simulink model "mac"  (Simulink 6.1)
settings: Solver=ode45  StartTime=0.0  StopTime=10  RelTol=1e-3
undefined symbols (not defined in the file or in its folder): coef, Ft, juan2, mac_clk_wrapper, netlist, XFix
libraries: xbsIndex_r3 x9

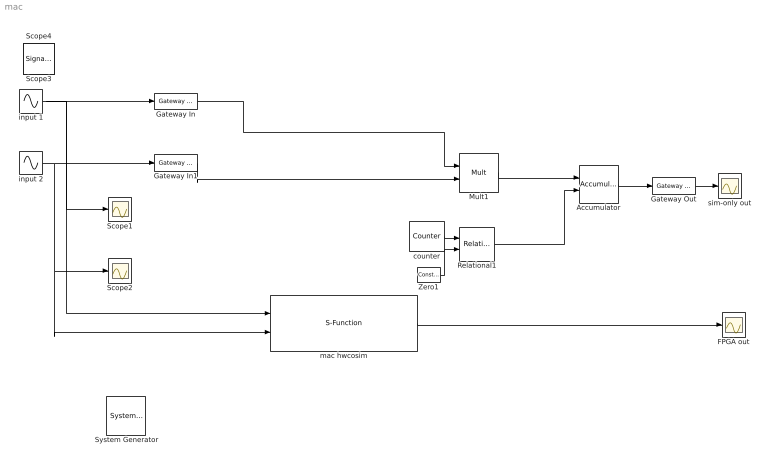
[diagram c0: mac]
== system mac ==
  " System Generator" : xbsIndex_r3/ System Generator  Tag=genX  xilinxfamily=Virtex2  part=xc2v1000  speed=-4  package=fg456  synthesis_tool=XST  directory=./netlist  testbench=off  simulink_period=1/2  sysclk_period=10  incr_netlist=off  trim_vbits=Everywhere in SubSystem  dbl_ovrd=According to Block Masks  core_generation=According to Block Masks  run_coregen=off  deprecated_control=off  eval_field=0
  Accumulator : xbsIndex_r3/Accumulator  n_bits=16  overflow=Wrap  operation=Add  scale=1  explicit_period=off  period=1  rst=on  hasbypass=off  en=off  dbl_ovrd=off  show_param=on  gen_core=off  use_rpm=on
  FPGA out : Scope
  Gateway In : xbsIndex_r3/Gateway In  arith_type="Signed  (2's comp)"  n_bits=8  bin_pt=6  quantization=Truncate  overflow=Wrap  period=1  timing_constraint=None  locs_specified=off  LOCs={}  needs_fixed_name=off  dbl_ovrd=off  show_param=off
  Gateway In1 : xbsIndex_r3/Gateway In  arith_type="Signed  (2's comp)"  n_bits=8  bin_pt=6  quantization=Truncate  overflow=Wrap  period=1  timing_constraint=None  locs_specified=off  LOCs={}  needs_fixed_name=off  dbl_ovrd=off  show_param=off
  Gateway Out : xbsIndex_r3/Gateway Out  output_type=Double  nbits=8  bin_pt=6  arith_type=Boolean  quantization=Truncate  overflow=Wrap  hdl_port=on  timing_constraint=None  locs_specified=off  LOCs={}  needs_fixed_name=off  show_param=off
  Mult1 : xbsIndex_r3/Mult  precision=Full  arith_type="Signed  (2's comp)"  n_bits=8  bin_pt=2  quantization=Truncate  overflow=Wrap  latency=2  explicit_period=on  period=1  en=off  dbl_ovrd=off  show_param=off  mult_type=Parallel  oversample=2  use_embedded=off  pipeline=on  use_rpm=on  placement_style=Rectangular Shape  gen_core=off
  Relational1 : xbsIndex_r3/Relational  mode=a=b  latency=0  explicit_period=on  period=-1  en=off  dbl_ovrd=off  show_param=off
  Scope1 : Scope
  Scope2 : Scope
  Zero1 : xbsIndex_r3/Constant  Priority=5  const=32  equ=P=C  arith_type=Unsigned  n_bits=5  bin_pt=0  opselect=C  inp2=PCIN>>17  opr=+  inp1=P  carry=CIN  iostate=0  explicit_period=off  period=Ft/length(coef)  dbl_ovrd=off
  counter : xbsIndex_r3/Counter  Priority=5  cnt_type=Count Limited  n_bits=5  bin_pt=0  arith_type=Unsigned  start_count=0  cnt_to=31  cnt_by_val=1  operation=Up  explicit_period=off  period=1  load_pin=off  rst=off  en=off  dbl_ovrd=off  show_param=off  use_rpm=on  gen_core=on
  input 1 : Sin  Amplitude=.5  Frequency=2*pi/23  Phase=pi/6  SampleTime=1
  input 2 : Sin  Amplitude=.5  Frequency=2*pi/23  Phase=pi/6  SampleTime=1
  mac hwcosim : S-Function  FunctionName=xlcosim  Parameters=sfcn_mwsv__  mask(Xilinx JTAG Hardware Co-Simulation){bitfileName=t:\juan2\netlist\mac_clk_wrapper.bit, clkSrc=Single Stepped, hasBufgmux=on, blkPeriod=0.5, IRLengths=[8,6], bscanPos=2, prtSignalType=XFix, prtNames={'gateway_in','gateway_in1','gateway_out'}, prtTypes={'Fix_8_6','Fix_8_6','Fix_16_12'}, prtDirs=[0,0,1], prtDataRates=[2,2,2]}
      mask prompts: bitfileName "Bit File Name"; clkSrc "Clock"; hasBufgmux "Supports BUFGMUX"; blkPeriod "Internal Block Period"; IRLengths "Instruction Reg Lengths"; bscanPos "BSCAN Position"; prtSignalType "Port Signal Type"; prtNames "Port Names (specified as cell array of strings)"; prtTypes "Port Types (specified as cell array of strings, eg 'Fix_8_7')"; prtDirs "Port Directions (specified as vector of integers, eg 'in'= 0 'out'=1)"; prtDataRates "Port Data Rates (specified as vector of integers)"
      mask help: Performs hardware co-simulation using JTAG and the Parallel Cable IV.
      mask init:
      | [bg,fg] = xlcmap('XBlock',1);
      | 
      | iPos = get_param(gcb,'Position');
      | iWidth=iPos(3)-iPos(1); iHeight=iPos(4)-iPos(2);
      | iCx=iWidth/2;
      | iCy=iHeight/2;
      | [logoX, logoY] = xlogo(iPos);
      | 
      | % support optional port that allows 
      | % selection between single-stepped and 
      | % free-running clocks during simulation
      | if (clkSrc == 3) 
      |   clkselprt = length(prtDirs)-sum(prtDirs)+1;
      |   clkseldir = 'input';
      |   clkselstr = 'clk_sel';
      | else
      |   clkselstr = '';
      |   if (length(prtDirs) == sum(prtDirs))
      |     clkseldir = 'output';
      |   else
      | 	clkseldir = 'input';
      |   end
      |   clkselprt = 1;
      | end
      | 
      | % assumes the cosim DLL resides in the same
      | % directory as the library containing the
      | % cosim block
      | libDir = which('JTAGRunTimeCosim');
      | binDir = fileparts(libDir);
      | 
      | % Extract target directory from bitstream
      | % name.
      | [targetDir,toplevelName] = fileparts(bitfileName);
      | 
      | % cosim DLL name goes here
      | engineDll = 'JTAGCosimEngine.dll';
      | 
      | % pass all mask workspace variables 
      | % to S-function
      | sfcn_mwsv__ = get_param(gcb, 'MaskWSVariables');
  sim-only out : Scope
  Scope3 : SignalViewerScope  IOType=viewer  RefreshTime=0.035000
  Scope4 : SignalViewerScope  IOType=viewer  RefreshTime=0.035000
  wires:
  Gateway Out/1 -> sim-only out/1
  input 1/1 -> Scope1/1, Gateway In/1, mac hwcosim/1
  input 2/1 -> Gateway In1/1, mac hwcosim/2, Scope2/1
  Mult1/1 -> Accumulator/1
  Accumulator/1 -> Gateway Out/1
  counter/1 -> Relational1/1
  Zero1/1 -> Relational1/2
  Relational1/1 -> Accumulator/2
  Gateway In/1 -> Mult1/1
  mac hwcosim/1 -> FPGA out/1
  Gateway In1/1 -> Mult1/2
